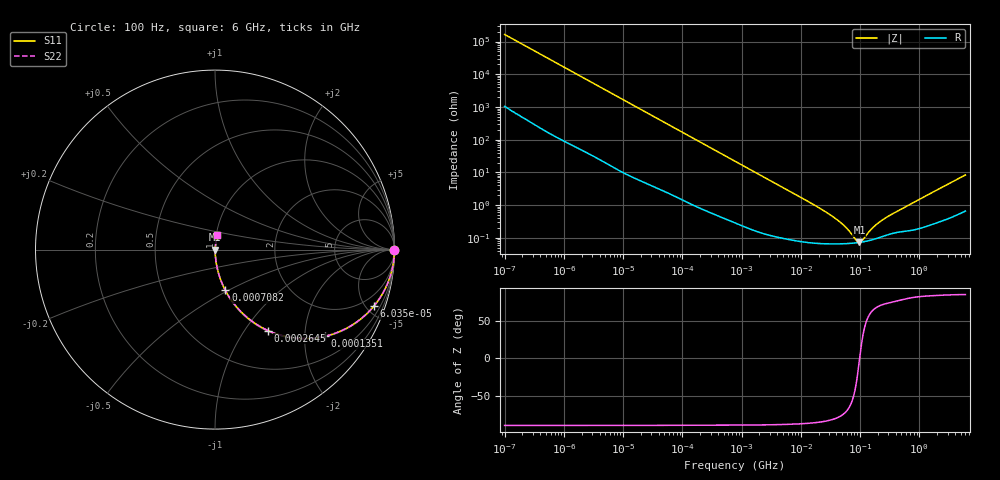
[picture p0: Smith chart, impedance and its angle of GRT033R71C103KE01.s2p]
!Murata Part Number: GRT033R71C103KE01
!These Parameters are Measured in Series Mode Connection
!Data Generated on Jun 19, 2026
!  o--ll--o
!Port1  Port2
!  o------o
!Operation Temp=25[degC], DC Bias Voltage=0[V]
!Freq. Start=100[Hz] Stop=6[GHz] 401[Steps]
# Hz S RI R 50
!Freq.(Hz) S11(Real) S11(Imag) S21(Real) S21(Imag) S12(Real) S12(Imag) S22(Real) S22(Imag)
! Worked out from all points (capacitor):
!   401 points, 100 Hz to 6 GHz, reference 50 ohm
!   read as one part in series: C = 9.63 nF near 109 Hz
!   lowest |Z| = 72.5 mohm at 97.54 MHz (marker M1)
!   series resonance near 98.34 MHz, so ESL is about 270 pH
!   S11 on the Smith chart (normalised r, x): 100 Hz: open; 60.35 kHz: 1.04, -5.60; 135.1 kHz: 1.02, -2.51; 264.5 kHz: 1.01, -1.29; 708.2 kHz: 1.01, -0.48; 6 GHz: 1.01, +0.17
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100  1 -0.000606  4.2e-06 0.000606  4.2e-06 0.000606  1 -0.000606
2008  0.9998 -0.012  0.000215 0.012  0.000215 0.012  0.9998 -0.012
12041  0.9945 -0.0713  0.00554 0.0713  0.00554 0.0713  0.9945 -0.0713
40335  0.9444 -0.2255  0.0556 0.2255  0.0556 0.2255  0.9444 -0.2255
60352  0.8849 -0.3152  0.1151 0.3152  0.1151 0.3152  0.8849 -0.3152
90302  0.7766 -0.4124  0.2234 0.4124  0.2234 0.4124  0.7766 -0.4124
135116  0.6109 -0.4832  0.3891 0.4832  0.3891 0.4832  0.6109 -0.4832
184852  0.4584 -0.4937  0.5416 0.4937  0.5416 0.4937  0.4584 -0.4937
264476  0.2948 -0.451  0.7052 0.451  0.7052 0.451  0.2948 -0.451
413847  0.1482 -0.3498  0.8518 0.3498  0.8518 0.3498  0.1482 -0.3498
708247  0.0578 -0.2272  0.9422 0.2272  0.9422 0.2272  0.0578 -0.2272
774597  0.0492 -0.2098  0.9508 0.2098  0.9508 0.2098  0.0492 -0.2098
2594782  0.00566 -0.0661  0.9943 0.0661  0.9943 0.0661  0.00566 -0.0661
1.555665e7  0.000814 -0.0109  0.9992 0.0109  0.9992 0.0109  0.000814 -0.0109
4.35672e7  0.000664 -0.00322  0.9993 0.00322  0.9993 0.00322  0.000664 -0.00322
5.960426e7  0.00067 -0.00185  0.9993 0.00185  0.9993 0.00185  0.00067 -0.00185
8.527865e7  0.000702 -0.000504  0.9993 0.000504  0.9993 0.000504  0.000702 -0.000504
9.753859e7  0.000724 -2.81e-05  0.9993 2.81e-05  0.9993 2.81e-05  0.000724 -2.81e-05
1.115611e8  0.000753 0.000443  0.9992 -0.000443  0.9992 -0.000443  0.000753 0.000443
1.825626e8  0.000939 0.00225  0.9991 -0.00225  0.9991 -0.00225  0.000939 0.00225
3.124326e8  0.0013 0.0046  0.9987 -0.0046  0.9987 -0.0046  0.0013 0.0046
6e9  0.0133 0.0818  0.9867 -0.0818  0.9867 -0.0818  0.0133 0.0818
